FUNCTION_BLOCK random
VAR_INPUT
	start: BOOL;
	Seed: INT:=50;
	stop: BOOL;

END_VAR

VAR_OUTPUT
	buffer : ARRAY [0..65535]OF UINT;
	data: UINT:=1;
END_VAR
VAR
	DRAND1: DRAND;
	Num: LREAL;
	Ftirg:F_TRIG;
	counter: UINT;
END_VAR

Ftirg(CLK:=stop , Q=> );




IF  start AND NOT Ftirg.Q THEN
	DRAND1(Seed:= Seed, Num=>Num );    (*Seed随便填，如果一个程序中使用多个DRAND，那么每个Seed就设为不同的数，产生的随机数也会不同*)
	data:=REAL_TO_UINT(5*Num+1);     (* 产生一个1-6之间的随机整数*)
	
	IF counter < 0 OR counter > 65535 THEN
		counter:= 0;
	END_IF	  
		
	buffer[counter] := data;

	counter:= counter + 1;
END_IF

END_FUNCTION_BLOCK
